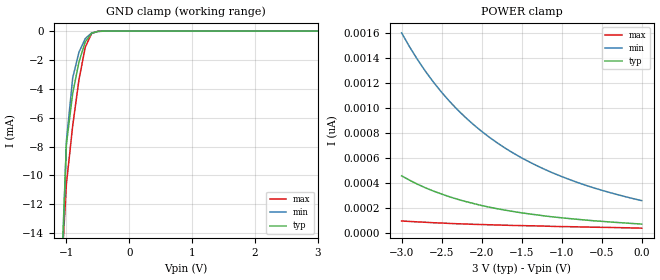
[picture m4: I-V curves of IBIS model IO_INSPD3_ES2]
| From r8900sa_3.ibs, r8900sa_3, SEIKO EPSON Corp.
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[Model]   IO_INSPD3_ES2
Model_type Input
Enable Active-Low
Polarity Non-Inverting
Vinh=2.4
Vinl=0.6
C_comp   2.5p   2p   3p
[Temperature Range] 25   85   -40
[Voltage Range]   3.0   2.7   3.3
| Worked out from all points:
|   GND clamp passes 1 mA (typ) near -0.72 V on its own axis
[GND Clamp]
-3V       -391.1mA   -327.5mA   -491.6mA
-1.1V     -19.18mA   -20.8mA    -18.4mA
-1V       -7.855mA   -7.614mA   -10.6mA
-900mV    -4.308mA   -3.239mA   -6.564mA
-800mV    -2.131mA   -1.46mA    -3.357mA
-700mV    -747.4uA   -523.1uA   -1.119mA
-600mV    -155uA     -130.4uA   -169.7uA
-500mV    -23.23uA   -25.44uA   -15.75uA
-400mV    -3.177uA   -4.273uA   -1.427uA
3V        73.56pA    308.2pA    37.29pA
[POWER Clamp]
-3V       458.8pA    1.6nA      98.23pA
-2.8V     391.3pA    1.386nA    90.95pA
-2.7V     362.4pA    1.291nA    87.99pA
-2.5V     313.3pA    1.126nA    81.85pA
-2.4V     291.2pA    1.053nA    78.67pA
-2.2V     253.6pA    923.8pA    74.35pA
-2V       221.6pA    813.8pA    69.8pA
-1.8V     195.5pA    719.6pA    66.05pA
-1.4V     154.3pA    568.3pA    59.91pA
-1V       123.6pA    453pA      53.32pA
-600mV    99.93pA    362.8pA    48.54pA
0V        73.56pA    260.9pA    40.93pA
